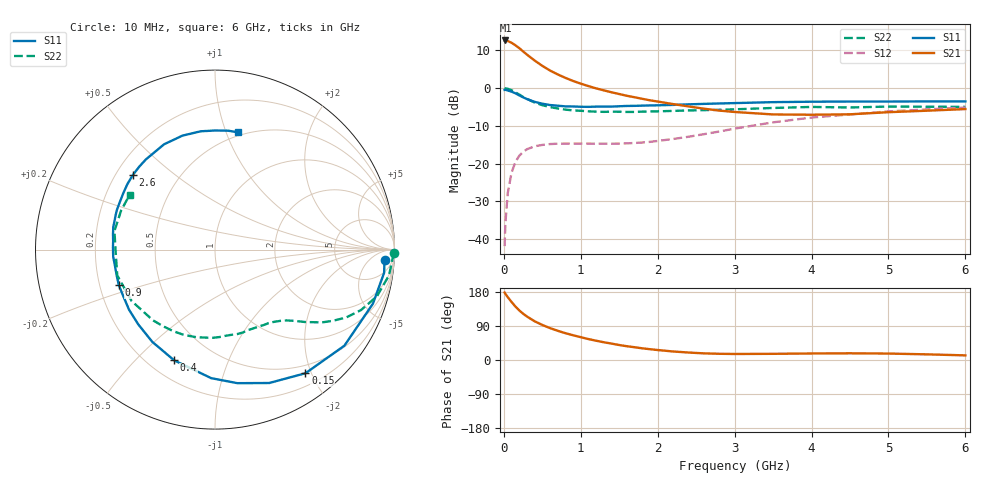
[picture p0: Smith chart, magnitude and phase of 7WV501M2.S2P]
! Infineon Technologies  Discrete & RF Semiconductors
! BFS17W
! Si NPN RF Bipolar Junction Transistor in SOT323
! VCE = 0.5 V  IC = 1.2 mA
! Common Emitter S-Parameters:  August  1999
# GHz  S  MA  R  50
!  f  S11  S21  S12  S22
! GHz  MAG  ANG  MAG  ANG  MAG  ANG  MAG  ANG
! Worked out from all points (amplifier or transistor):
!   36 points, 10 MHz to 6 GHz, reference 50 ohm
!   highest |S21| = 12.6 dB at 20 MHz (marker M1)
!   |S21| within 3 dB of that: start of sweep to 256.1 MHz
!   unconditionally stable (mu >= 1): 839.3 MHz to end of sweep
!   at 250 MHz: K = 0.33, MSG = 13.3 dB, |S12| = -16.9 dB
!   at 1.4 GHz: K = 1.45, MAG = 2.8 dB, |S12| = -14.7 dB
!   at 6 GHz: K = 1.16, MAG = -2.6 dB, |S12| = -5.1 dB
!   S11 on the Smith chart (normalised r, x): 10 MHz: 16, -18; 150 MHz: 0.38, -1.91; 400 MHz: 0.30, -0.65; 900 MHz: 0.28, -0.17; 2.6 GHz: 0.27, +0.36; 6 GHz: 0.47, +1.10
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0.01  0.9463 -3.6  4.255 178.0  0.0081 86.9  0.9976 -1.2
0.02  0.9511 -7.8  4.268 174.6  0.016 85.0  0.9894 -3.3
0.05  0.93 -18.9  4.2 166.1  0.0403 78.5  0.9804 -8.4
0.1  0.898 -36.6  3.979 153.3  0.076 68.6  0.9388 -16.1
0.15  0.8536 -53.8  3.687 141.2  0.1051 58.5  0.8804 -22.5
0.2  0.8023 -67.9  3.38 131.0  0.1271 51.8  0.8225 -27.4
0.25  0.7545 -80.5  3.057 122.3  0.1429 45.1  0.7649 -31.3
0.3  0.7165 -91.7  2.776 114.8  0.1552 40.7  0.7197 -34.3
0.4  0.6577 -110.2  2.317 102.2  0.1698 33.3  0.6438 -38.8
0.5  0.6215 -124.2  1.969 92.5  0.177 28.8  0.5947 -41.9
0.6  0.597 -135.7  1.708 84.2  0.1817 25.7  0.561 -44.7
0.7  0.5845 -145.0  1.518 77.1  0.1837 23.9  0.5373 -47.7
0.9  0.5713 -159.7  1.242 65.3  0.1846 21.8  0.5068 -53.9
1.1  0.5648 -171.3  1.062 55.2  0.1844 22.0  0.4926 -60.6
1.6  0.5806 167.5  0.791 36.3  0.1857 27.2  0.4835 -79.3
2.2  0.5992 148.8  0.614 22.5  0.2121 37.8  0.4991 -102.1
2.6  0.6182 137.8  0.534 17.5  0.2455 42.2  0.5105 -117.2
3.5  0.6517 115.8  0.448 16.3  0.3521 41.7  0.5457 -148.3
4  0.6604 105.9  0.444 17.2  0.4079 37.0  0.5633 -165.2
4.5  0.6639 96.9  0.45 17.7  0.4475 31.9  0.554 -179.5
5.5  0.6666 83.7  0.502 14.9  0.5224 22.3  0.5666 157.3
6  0.6661 78.7  0.528 12.2  0.5533 17.5  0.5649 147.2
